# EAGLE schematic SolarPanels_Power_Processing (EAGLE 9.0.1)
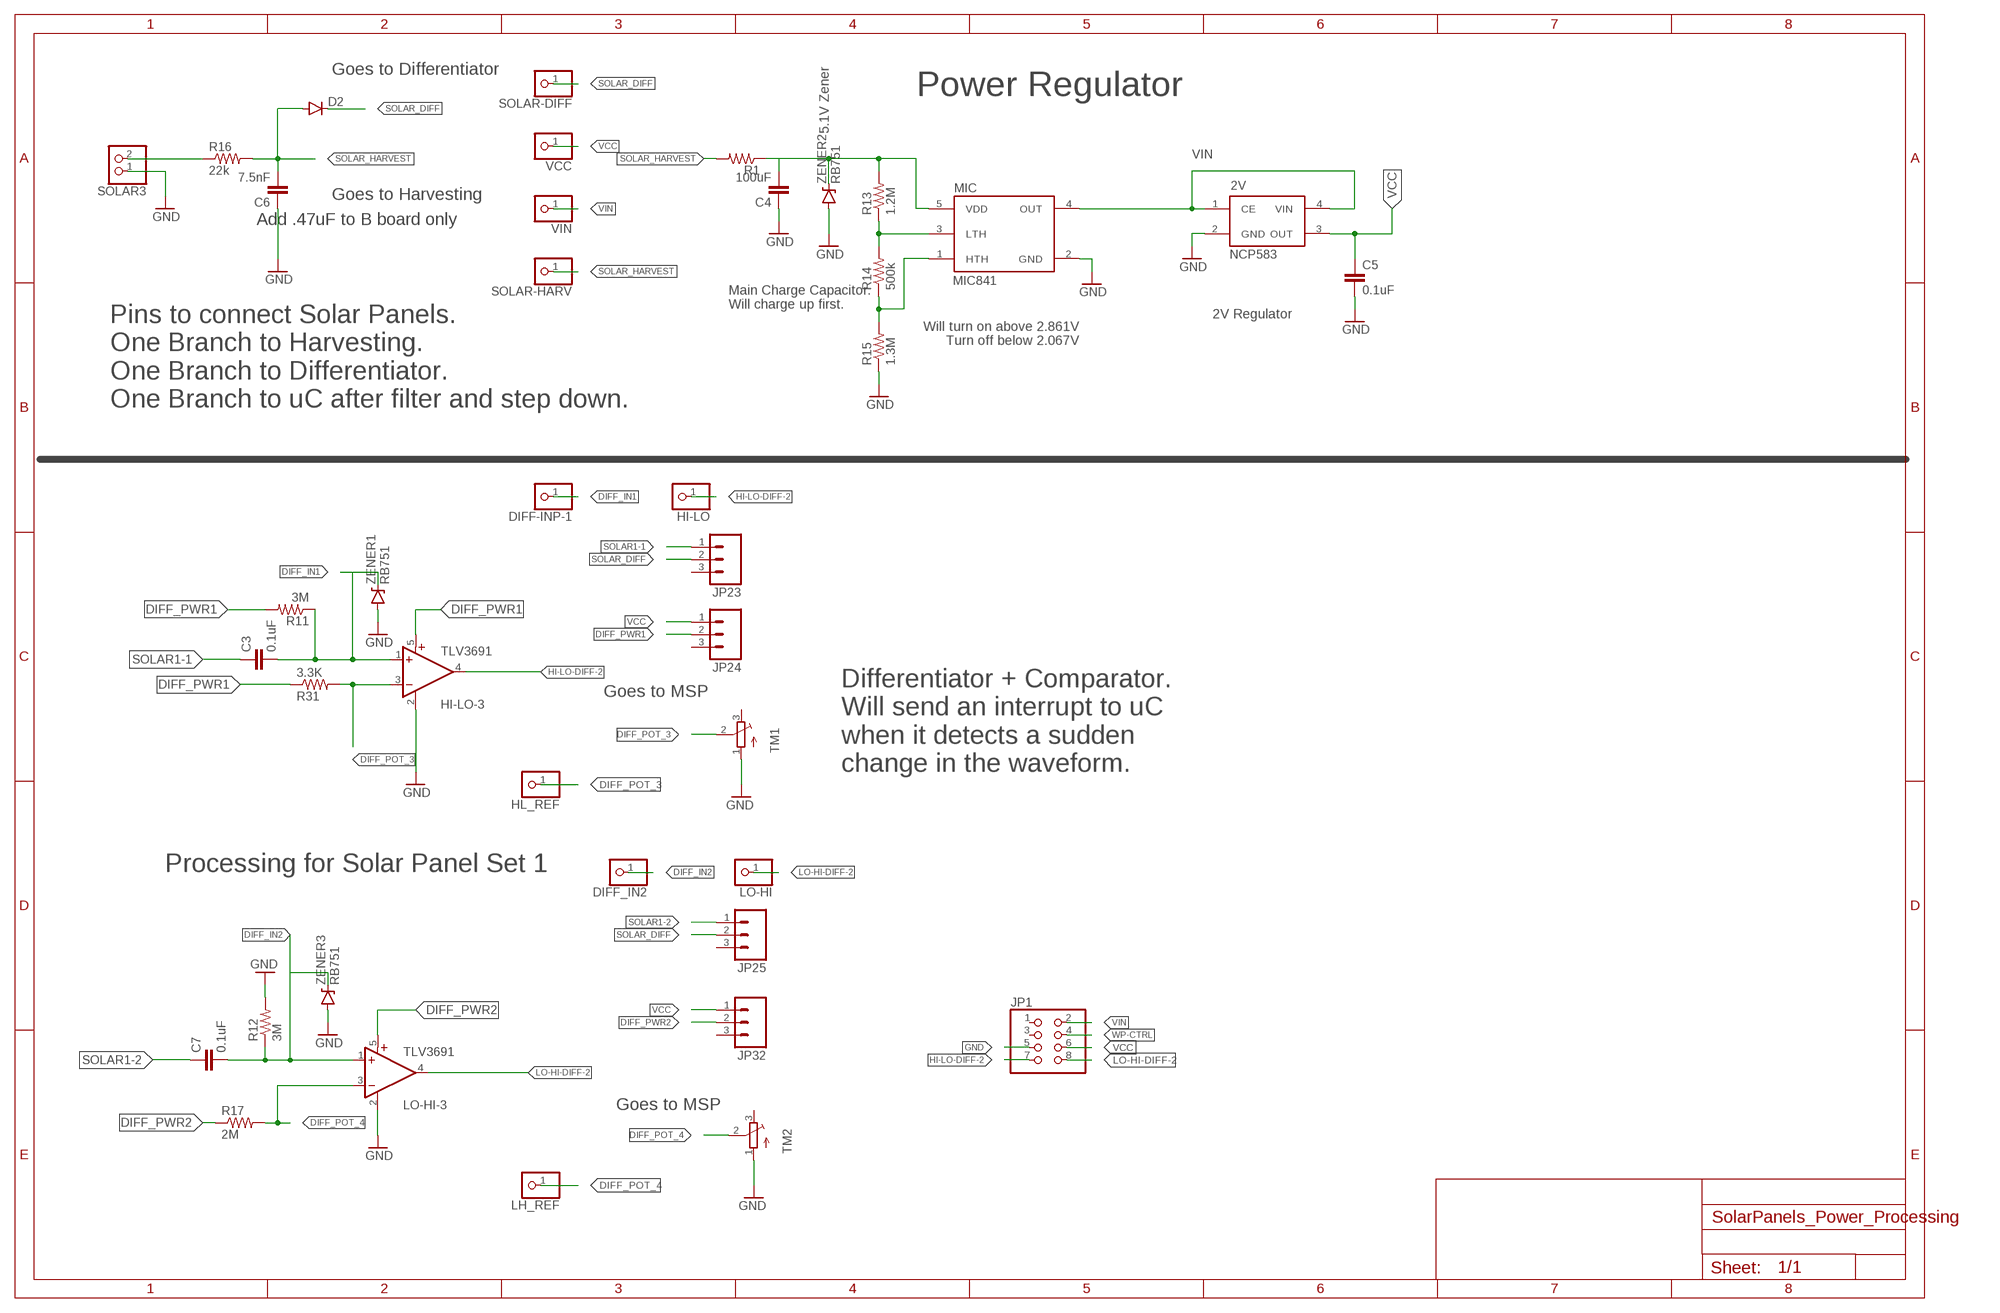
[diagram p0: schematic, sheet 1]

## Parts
2V  NCP583  [SC82-AB_1PRIMARY]
3.3K  R31  RESISTOR0805-RES  [0805]
C3  0.1uF  CAP0805  [0805]
C4  100uF  CAP0805  [0805]
C5  0.1uF  CAP0805  [0805]
C6  7.5nF  CAP0805  [0805]
C7  0.1uF  CAP0805  [0805]
D2  DIODESOD523  [SOD523]
DIFF-INP-1  PINHD-1X1  [1X01]
DIFF_IN2  PINHD-1X1  [1X01]
HI-LO  PINHD-1X1  [1X01]
HI-LO-3  TLV3691  [SC70-5]
HL_REF  PINHD-1X1  [1X01]
JP1  PINHD-2X4/90  [2X04/90]
JP23  M03  [1X03-1.27MM]
JP24  M03  [1X03-1.27MM]
JP25  M03  [1X03-1.27MM]
JP32  M03  [1X03-1.27MM]
LH_REF  PINHD-1X1  [1X01]
LO-HI  PINHD-1X1  [1X01]
LO-HI-3  TLV3691  [SC70-5]
MIC  MIC841  [SC70-5]
R1  RESISTOR0805-RES  [0805]
R11  3M  RESISTOR0805-RES  [0805]
R12  3M  RESISTOR0805-RES  [0805]
R13  1.2M  RESISTOR0805-RES  [0805]
R14  500k  RESISTOR0805-RES  [0805]
R15  1.3M  RESISTOR0805-RES  [0805]
R16  22k  RESISTOR0805-RES  [0805]
R17  2M  RESISTOR0805-RES  [0805]
SOLAR3  PINHD-1X2  [1X02]
SOLAR-DIFF  PINHD-1X1  [1X01]
SOLAR-HARV  PINHD-1X1  [1X01]
TM1  TRIMPOTTC33X  [TC33X]
TM2  TRIMPOTTC33X  [TC33X]
VCC  PINHD-1X1  [1X01]
VIN  PINHD-1X1  [1X01]
ZENER1  RB751  DIODE-ZENER  [SOD-523]
ZENER2  RB751  DIODE-ZENER  [SOD-523]
ZENER3  RB751  DIODE-ZENER  [SOD-523]

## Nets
DIFF_IN1: C3.2 DIFF-INP-1.1 HI-LO-3.1(+IN) R11.1 ZENER1.CATHODE(C)
DIFF_IN2: C7.2 DIFF_IN2.1 LO-HI-3.1(+IN) R12.1 ZENER3.CATHODE(C)
DIFF_POT_3: 3.3K.2 HI-LO-3.3(-IN) HL_REF.1 TM1.2(S)
DIFF_POT_4: LH_REF.1 LO-HI-3.3(-IN) R17.2 TM2.2(S)
DIFF_PWR1: 3.3K.1 HI-LO-3.5(V+) JP24.2 R11.2
DIFF_PWR2: JP32.2 LO-HI-3.5(V+) R17.1
GND: 2V.2(GND) C4.1 C5.2 C6.1 HI-LO-3.2(GND) JP1.5 LO-HI-3.2(GND) MIC.2(GND) R12.2 R15.1 SOLAR3.1 TM1.1(A) TM2.1(A) ZENER1.ANODE(A) ZENER2.ANODE(A) ZENER3.ANODE(A)
HI-LO-DIFF-2: HI-LO-3.4(OUT) HI-LO.1 JP1.7
LO-HI-DIFF-2: JP1.8 LO-HI-3.4(OUT) LO-HI.1
MIC_INPUT: C4.2 MIC.5(VDD) R1.1 R13.2 ZENER2.CATHODE(C)
N$11: MIC.3(LTH) R13.1 R14.2
N$12: MIC.1(HTH) R14.1 R15.2
SOLAR1: R16.1 SOLAR3.2
SOLAR1-1: C3.1 JP23.1
SOLAR1-2: C7.1 JP25.1
SOLAR_DIFF: D2.C JP23.2 JP25.2 SOLAR-DIFF.1
SOLAR_HARVEST: C6.2 D2.A R1.2 R16.2 SOLAR-HARV.1
VCC: 2V.3(OUT) C5.1 JP1.6 JP24.1 JP32.1 VCC.1
VIN: 2V.1(CE) 2V.4(VIN) JP1.2 MIC.4(OUT) VIN.1
WP-CTRL: JP1.4
Unconnected: JP1.1 JP1.3 JP23.3 JP24.3 JP25.3 JP32.3 TM1.3(E) TM2.3(E)

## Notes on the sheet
- Goes to Differentiator
- Power Regulator
- 5.1V Zener
- Goes to Harvesting
- Add .47uF to B board only
- Main Charge Capacitor.
  Will charge up first.
- 2V Regulator
- Will turn on above 2.861V
  Turn off below 2.067V
- Pins to connect Solar Panels.
  One Branch to Harvesting.
  One Branch to Differentiator.
  One Branch to uC after filter and step down.
- Goes to MSP
- Differentiator + Comparator.
  Will send an interrupt to uC 
  when it detects a sudden 
  change in the waveform.
- Processing for Solar Panel Set 1
- Goes to MSP

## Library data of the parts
2V = ncp583:NCP583: NCP583 - Ultra-Low Iq 150 mA CMOS LDO Regulator with Enable The NCP583 series of low dropout regulators are designed for portable battery powered applications which require precise output voltage accuracy and low quiescent current. These devices feature an enable function which lowers current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
3.3K R1 R11-R17 = SparkFun-Resistors:RESISTOR: Resistor
C3-C7 = SparkFun-Capacitors:CAP: Capacitor
D2 = SparkFun-DiscreteSemi:DIODE: Diode
DIFF-INP-1 DIFF_IN2 HI-LO HL_REF LH_REF LO-HI SOLAR-DIFF SOLAR-HARV VCC VIN = adafruit:PINHD-1X1: Pin header 1x1 for 0.1" spacing
HI-LO-3 LO-HI-3 = fedpower:TLV3691: 0.9-V to 6.5-V, Nanopower Comparator Datasheets Analog Signal Chain Guide TLV3691 Manufacturer Product Page TLV3691IDPFR Specifications Standard Package 1 CategoryIntegrated Circuits (ICs) FamilyLinear - Comparators Series- Packaging Cut Tape (CT) TypeGeneral Purpose Number of Elements1 Output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
JP1 = pinhead:PINHD-2X4: PIN HEADER
JP23-JP25 JP32 = SparkFun-Connectors:M03: Header 3 Standard 3-pin 0.1" header. Use with straight break away headers (SKU : PRT-00116), right angle break away headers (PRT-00553), swiss pins (PRT-00743), machine pins (PRT-00117), and female headers (PRT-00115). Molex polarized connector foot print use with SKU : PRT-08232 with associated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
MIC = mic841:MIC841: MIC841:Comparator with reference and adj. hysteresis
SOLAR3 = pinhead:PINHD-1X2: PIN HEADER
TM1 TM2 = adafruit:TRIMPOT: SMT trimmer potentiometer part number TC33X http://www.ladyada.net/library/eagle
ZENER1-ZENER3 = Parts:DIODE-ZENER: Zener Diode

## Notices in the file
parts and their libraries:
SparkFun-Capacitors: Licensing: Creative Commons ShareAlike 4.0 International - https://creativecommons.org/licenses/by-sa/4.0
